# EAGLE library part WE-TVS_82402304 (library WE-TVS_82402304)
TVS Diode Array WE-TVS, Standard Series - Low capazity - No leakage current - Low clamping voltage - high ESD voltage protection - Uni- and bidirectional protection -- DC Distribution -- Headsets and Accessoires -- PDAs -- Digital Cameras -- MP3-Players -- Touch Panels
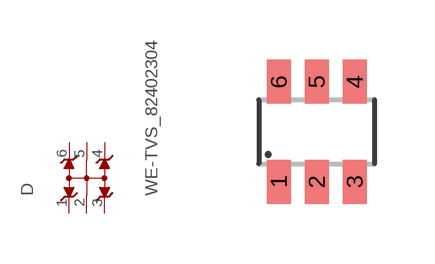
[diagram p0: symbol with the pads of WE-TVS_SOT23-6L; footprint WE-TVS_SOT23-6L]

Designator prefix D

## WE-TVS_82402304 (MPN: 82402304; OC_FARNELL: 1825865; OC_NEWARK: 79R6954; PACKAGE: SOT23-6L; SUPPLIER: Wuerth Elektronik)  [WE-TVS_SOT23-6L]
1  1  pas
2  GND  pwr
3  2  pas
4  3  pas
5  GND  pwr
6  4  pas

## Footprint WE-TVS_SOT23-6L (pad centres in mm)
TVS Diode Array WE-TVS
smd 0.6 x 1.1: 1 -0.95,-1.25; 2 0,-1.25; 3 0.95,-1.25; 4 0.95,1.25; 5 0,1.25; 6 -0.95,1.25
